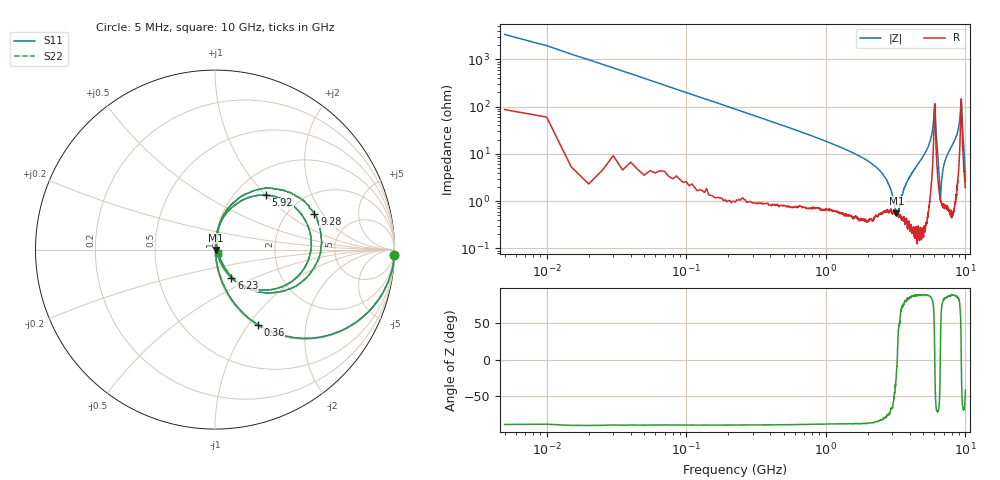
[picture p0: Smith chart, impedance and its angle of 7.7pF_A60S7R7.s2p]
! Amotech Co.,Ltd.
! http://www.amotech.co.kr/
! Part Number: A60S7R7
! These Parameters are Measured in Series Mode Connection
! Operation Temp=25[degC], DC Bias Voltage=0[V]
! Freq. Start=5[MHz] Stop=10[GHz], 2000[Steps]
! Date: Monday, July 13, 2020, 01:33:03
# GHZ S RI R 50.000000
!Freq.(Hz) S11(Real) S11(Imag) S21(Real) S21(Imag) S12(Real) S12(Imag) S22(Real) S22(Imag)
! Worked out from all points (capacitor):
!   2000 points, 5 MHz to 10 GHz, reference 50 ohm
!   read as one part in series: C = 7.99 pF near 55 MHz
!   lowest |Z| = 548 mohm at 3.205 GHz (marker M1)
!   series resonance near 3.251 GHz, so ESL is about 300 pH
!   S11 on the Smith chart (normalised r, x): 5 MHz: 3, -67; 360 MHz: 1.02, -1.10; 5.92 GHz: 1.37, +1.00; 6.23 GHz: 1.14, -0.37; 9.28 GHz: 2.74, +1.66; 10 GHz: 1.04, -0.03
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0.005  0.9984 -0.0296  0.00164 0.0296  0.00164 0.0296  0.9984 -0.0296
0.065  0.9007 -0.292  0.0993 0.292  0.0993 0.292  0.9007 -0.292
0.115  0.7466 -0.4294  0.2534 0.4294  0.2534 0.4294  0.7466 -0.4294
0.36  0.237 -0.4174  0.763 0.4174  0.763 0.4174  0.237 -0.4174
1.675  0.0135 -0.0936  0.9865 0.0936  0.9865 0.0936  0.0135 -0.0936
2.7  0.0067 -0.0287  0.9933 0.0287  0.9933 0.0287  0.0067 -0.0287
3.205  0.00513 -0.00184  0.9949 0.00184  0.9949 0.00184  0.00513 -0.00184
3.34  0.00486 0.00494  0.9951 -0.00494  0.9951 -0.00494  0.00486 0.00494
3.81  0.00418 0.0248  0.9958 -0.0248  0.9958 -0.0248  0.00418 0.0248
5.005  0.0101 0.0905  0.9899 -0.0905  0.9899 -0.0905  0.0101 0.0905
5.69  0.0656 0.2067  0.9344 -0.2067  0.9344 -0.2067  0.0656 0.2067
5.92  0.2845 0.3033  0.7155 -0.3033  0.7155 -0.3033  0.2845 0.3033
6.035  0.5334 -0.00747  0.4666 0.00747  0.4666 0.00747  0.5334 -0.00747
6.23  0.0919 -0.1572  0.9081 0.1572  0.9081 0.1572  0.0919 -0.1572
6.585  0.0113 -0.00497  0.9887 0.00497  0.9887 0.00497  0.0113 -0.00497
6.67  0.01 0.0118  0.99 -0.0118  0.99 -0.0118  0.01 0.0118
7.09  0.0119 0.0641  0.9881 -0.0641  0.9881 -0.0641  0.0119 0.0641
8.335  0.0404 0.1789  0.9596 -0.1789  0.9596 -0.1789  0.0404 0.1789
8.97  0.1583 0.3028  0.8417 -0.3028  0.8417 -0.3028  0.1583 0.3028
9.28  0.5538 0.1985  0.4462 -0.1985  0.4462 -0.1985  0.5538 0.1985
9.48  0.3232 -0.2401  0.6768 0.2401  0.6768 0.2401  0.3232 -0.2401
10  0.0193 -0.0165  0.9807 0.0165  0.9807 0.0165  0.0193 -0.0165
